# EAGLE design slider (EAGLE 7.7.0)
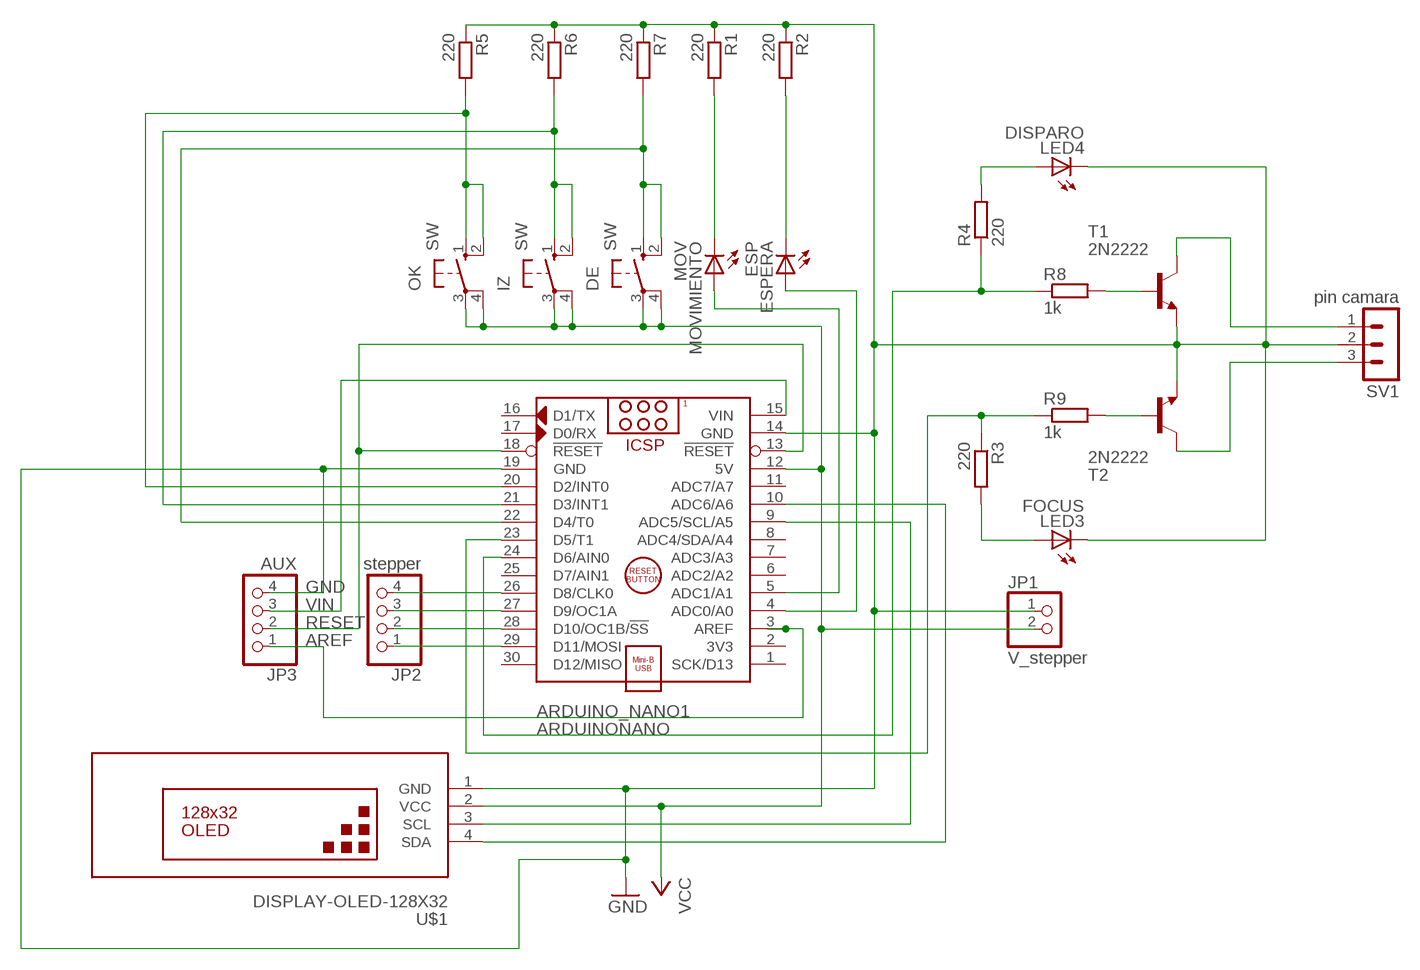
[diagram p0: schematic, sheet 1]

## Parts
ARDUINO_NANO1  ARDUINONANO  ARDUINO_NANO  [ARDUINO_NANO]
DE  SW  40-XX  [B3F-40XX]
ESPERA  ESP  LED5MM  [LED5MM]
IZ  SW  40-XX  [B3F-40XX]
JP1  V_stepper  PINHD-1X2  [1X02]
JP2  stepper  PINHD-1X4  [1X04]
JP3  AUX  PINHD-1X4  [1X04]
LED3  FOCUS  LED5MM  [LED5MM]
LED4  DISPARO  LED5MM  [LED5MM]
MOVIMIENTO  MOV  LED5MM  [LED5MM]
OK  SW  40-XX  [B3F-40XX]
R1  220  R-EU_0204/5  [0204/5]
R2  220  R-EU_0204/5  [0204/5]
R3  220  R-EU_0204/5  [0204/5]
R4  220  R-EU_0204/5  [0204/5]
R5  220  R-EU_0204/5  [0204/5]
R6  220  R-EU_0204/5  [0204/5]
R7  220  R-EU_0204/5  [0204/5]
R8  1k  R-EU_0204/5  [0204/5]
R9  1k  R-EU_0204/5  [0204/5]
SV1  pin camara  MA03-1  [MA03-1]
T1  2N2222  [TO92-EBC-OVAL]
T2  2N2222  [TO92-EBC-OVAL]
U$1  DISPLAY-OLED-128X32  [DISPLAY-OLED-128X32]

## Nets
AREF: ARDUINO_NANO1.3(AREF) JP3.1
GND: ARDUINO_NANO1.14(GND) ARDUINO_NANO1.19(GND) JP1.1 JP3.4 LED3.K(C) LED4.K(C) R1.1 R2.1 R5.1 R6.1 R7.1 SV1.2 T1.E T2.E U$1.1(GND)
N$1: ARDUINO_NANO1.24(D6/AIN0) R4.1 R8.1
N$2: ARDUINO_NANO1.29(D11/MOSI) JP2.1
N$3: ARDUINO_NANO1.28(D10/OC1B/!SS) JP2.2
N$4: ARDUINO_NANO1.27(D9/OC1A) JP2.3
N$5: MOVIMIENTO.K(C) R1.2
N$6: ESPERA.K(C) R2.2
N$7: ARDUINO_NANO1.22(D4/T0) DE.1(S) DE.2(S1) R7.2
N$8: R9.2 T2.B
N$9: R8.2 T1.B
N$10: LED4.A R4.2
N$12: ARDUINO_NANO1.4(ADC0/A0) ESPERA.A
N$13: LED3.A R3.2
N$14: SV1.3 T2.C
N$15: SV1.1 T1.C
N$16: ARDUINO_NANO1.23(D5/T1) R3.1 R9.1
N$17: ARDUINO_NANO1.5(ADC1/A1) MOVIMIENTO.A
N$18: ARDUINO_NANO1.21(D3/INT1) IZ.1(S) IZ.2(S1) R6.2
N$19: ARDUINO_NANO1.20(D2/INT0) OK.1(S) OK.2(S1) R5.2
N$21: ARDUINO_NANO1.9(ADC5/SCL/A5) U$1.3(SCL)
N$22: ARDUINO_NANO1.10(ADC6/A6) U$1.4(SDA)
N$23: ARDUINO_NANO1.26(D8/CLK0) JP2.4
RESET: ARDUINO_NANO1.13(!RESET) ARDUINO_NANO1.18(!RESET) JP3.2
VCC: ARDUINO_NANO1.12(5V) DE.3(P) DE.4(P1) IZ.3(P) IZ.4(P1) JP1.2 OK.3(P) OK.4(P1) U$1.2(VCC)
VIN: ARDUINO_NANO1.15(VIN) JP3.3
Unconnected: ARDUINO_NANO1.1(SCK/D13) ARDUINO_NANO1.2(3V3) ARDUINO_NANO1.6(ADC2/A2) ARDUINO_NANO1.7(ADC3/A3) ARDUINO_NANO1.8(ADC4/SDA/A4) ARDUINO_NANO1.11(ADC7/A7) ARDUINO_NANO1.16(D1/TX) ARDUINO_NANO1.17(D0/RX) ARDUINO_NANO1.25(D7/AIN1) ARDUINO_NANO1.30(D12/MISO)

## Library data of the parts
ARDUINO_NANO1 = ArduinoNanoV30:ARDUINO_NANO: Arduino Nano V3.0 Module Overview: The Arduino Nano is a small, complete, and breadboard-friendly board based on the ATmega328 (Arduino Nano 3.x) or ATmega168 (Arduino Nano 2.x). It has more or less the same functionality of the Arduino Duemilanove, but in a different package. It lacks only a DC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
DE IZ OK = switch-omron:40-XX: OMRON SWITCH; MF: OMRON COMPONENTS USA; MPN: B3F-4000; OC_FARNELL: 176434; OC_NEWARK: 36K3105
ESPERA LED3 LED4 MOVIMIENTO = adafruit:LED: LED
JP1 = pinhead:PINHD-1X2: PIN HEADER
JP2 JP3 = pinhead:PINHD-1X4: PIN HEADER
R1-R9 = rcl:R-EU_: RESISTOR, European symbol
SV1 = con-lstb:MA03-1: PIN HEADER; OC_FARNELL: unknown; OC_NEWARK: unknown
T1 T2 = adafruit:2N2222: NPN TRANSISTOR Big oval pads
U$1 = diy-modules:DISPLAY-OLED-128X32: 128x32 Dot Matrix OLED Module with I2C interface based on SSD1306 chip More details available here: http://www.tinyosshop.com/index.php?route=product/product&product_id=953 Schematic available here: http://www.tinyosshop.com/datasheet/OLED%2012832.pdf SSD1306 datasheet: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

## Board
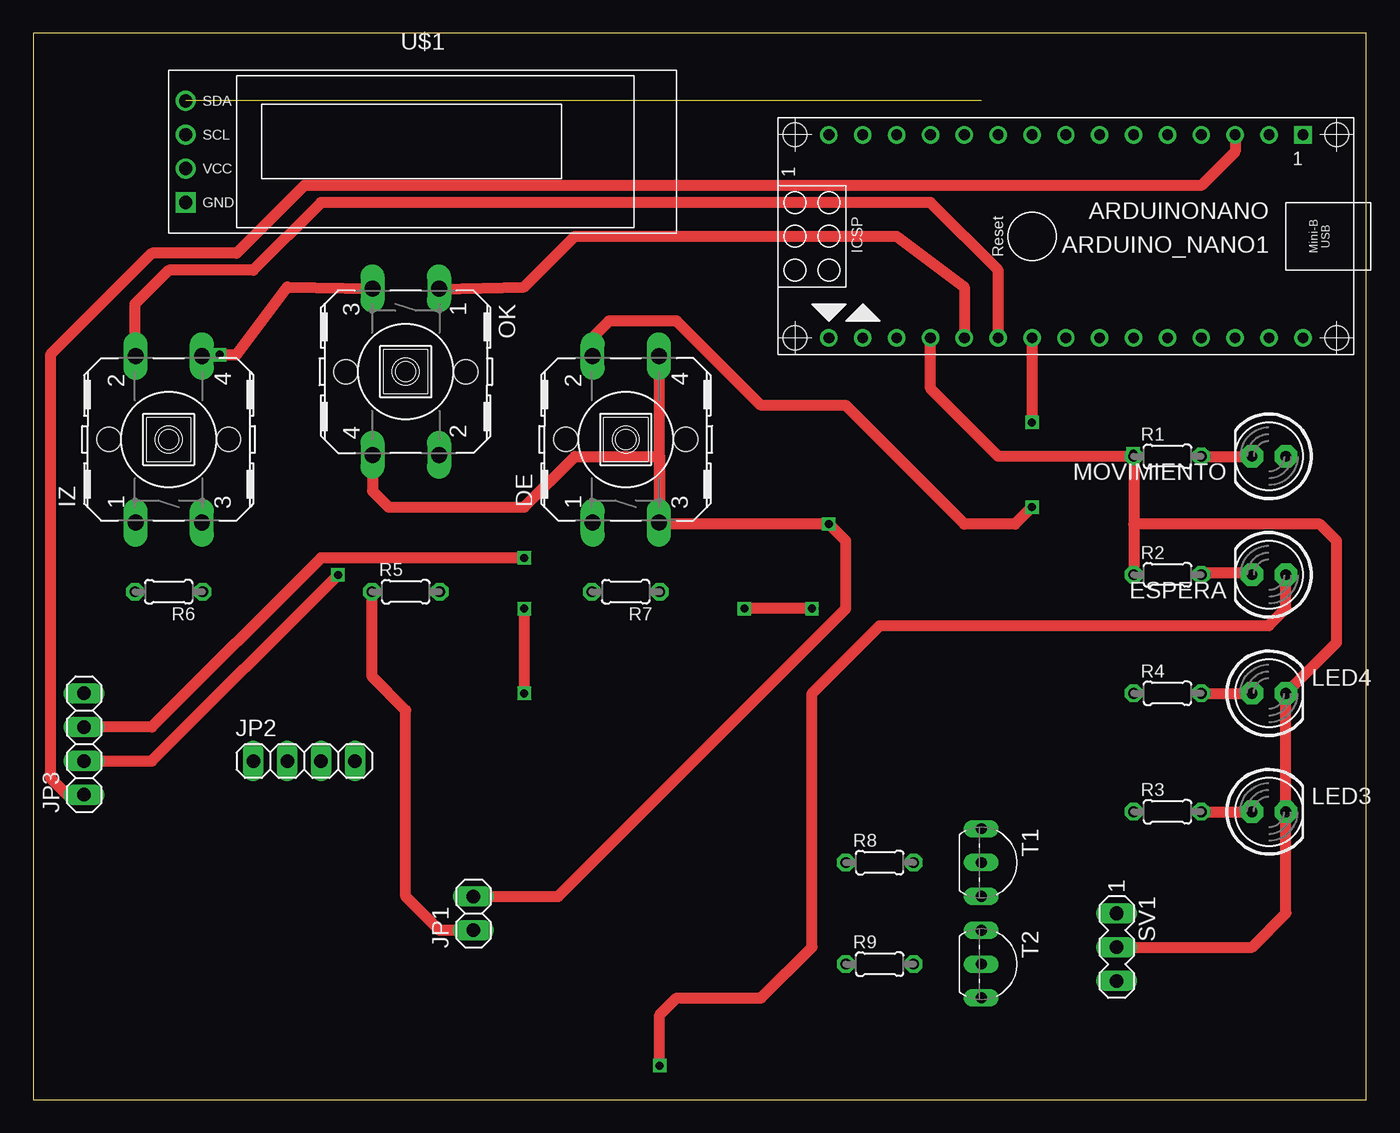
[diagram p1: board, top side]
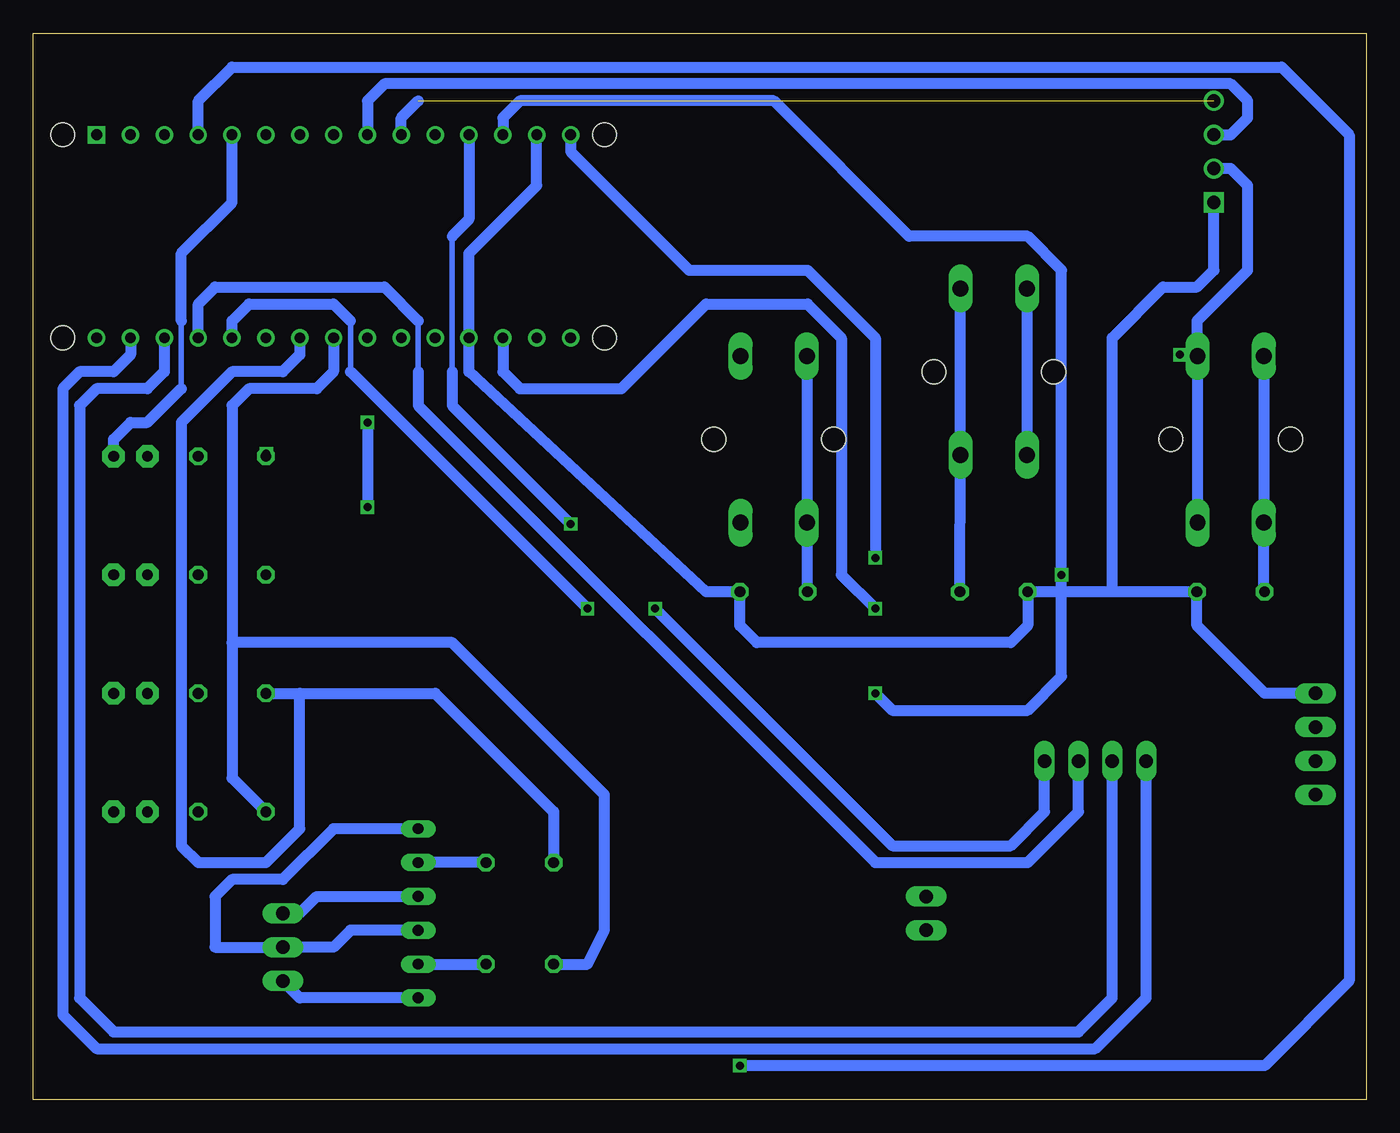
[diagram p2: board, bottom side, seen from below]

Size 100 x 80 mm. Coordinates in mm from the lower left corner, seen from the top.
Outline: 0,0 100,0 100,80 0,80 0,0
Copper layers (1*16): Top 0.035mm / dielectric 1.5mm / Bottom 0.035mm
Design rules "default": minimum track width 10mil, minimum drill 24mil, track to track 8mil, track to pad 8mil, pad to pad 8mil, via to via 8mil, smd to smd 8mil, copper to edge 40mil, drill to drill 8mil, minimum pad ring 10mil, minimum via ring 8mil, stop-mask expansion 4mil, vias tented up to drill 0mil, thermal gap 10mil

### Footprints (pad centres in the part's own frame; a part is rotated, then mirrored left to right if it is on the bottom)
ARDUINO_NANO = drill 0.8 square: 1 -20.32,-7.62 | drill 0.8: 2 -17.78,-7.62; 3 -15.24,-7.62; 4 -12.7,-7.62; 5 -10.16,-7.62; 6 -7.62,-7.62; 7 -5.08,-7.62; 8 -2.54,-7.62; 9 0,-7.62; 10 2.54,-7.62; 11 5.08,-7.62; 12 7.62,-7.62; 13 10.16,-7.62; 14 12.7,-7.62; 15 15.24,-7.62; 16 15.24,7.62; 17 12.7,7.62; 18 10.16,7.62; 19 7.62,7.62; 20 5.08,7.62; 21 2.54,7.62; 22 0,7.62; 23 -2.54,7.62; 24 -5.08,7.62; 25 -7.62,7.62; 26 -10.16,7.62; 27 -12.7,7.62; 28 -15.24,7.62; 29 -17.78,7.62; 30 -20.32,7.62 | hole 1.778: -22.86,-7.62; -22.86,7.62; 17.78,7.62; 17.78,-7.62
B3F-40XX = drill 1.194 long: 1 -6.248,2.489; 2 6.248,2.489; 3 -6.248,-2.489; 4 6.248,-2.489 | hole 1.803: 0,-4.496; 0,4.496
LED5MM = drill 0.813 pad 1.676 octagon: A -1.27,0; K 1.27,0
1X02 = drill 1.016 long: 1 -1.27,0; 2 1.27,0
1X04 = drill 1.016 long: 1 -3.81,0; 2 -1.27,0; 3 1.27,0; 4 3.81,0
0204/5 = drill 0.813 octagon: 1 -2.54,0; 2 2.54,0
MA03-1 = drill 1.016 long: 1 -2.54,0; 2 0,0; 3 2.54,0
TO92-EBC-OVAL = drill 0.813 long: B 0,-1.27; C 2.54,-1.27; E -2.54,-1.27
DISPLAY-OLED-128X32 = drill 1 square: 1 -17.78,-3.81 | drill 1: 2 -17.78,-1.27; 3 -17.78,1.27; 4 -17.78,3.81

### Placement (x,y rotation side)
ARDUINO_NANO1  74.93,64.77 180 top
DE  44.45,49.53 90 top
ESPERA  92.71,39.37 180 top
IZ  10.16,49.53 90 top
JP1  33.02,13.97 90 top
JP2  20.32,25.4 0 top
JP3  3.81,26.67 90 top
LED3  92.71,21.59 0 top
LED4  92.71,30.48 0 top
MOVIMIENTO  92.71,48.26 180 top
OK  27.94,54.61 270 top
R1  85.09,48.26 0 top
R2  85.09,39.37 0 top
R3  85.09,21.59 0 top
R4  85.09,30.48 0 top
R5  27.94,38.1 0 top
R6  10.16,38.1 180 top
R7  44.45,38.1 180 top
R8  63.5,17.78 0 top
R9  63.5,10.16 0 top
SV1  81.28,11.43 270 top
T1  72.39,17.78 270 top
T2  72.39,10.16 270 top
U$1  29.21,71.12 0 top

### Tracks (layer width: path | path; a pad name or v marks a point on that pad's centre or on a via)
AREF
  Top 0.813: ARDUINO_NANO1.3 90.17,71.12 87.63,68.58 20.32,68.58 15.24,63.5 8.89,63.5 1.27,55.88 1.27,24.13 2.54,22.86 JP3.1
GND  (via drill 0.6)
  Top 0.813: JP1.1 30.48,12.7 27.94,15.24 27.94,29.21 25.4,31.75 R5.1 | SV1.2 91.44,11.43 93.98,13.97 LED3.K LED4.K 97.79,34.29 97.79,41.91 96.52,43.18 82.55,43.18 R2.1 R1.1 | v82.53,48.46 82.32,48.26 72.39,48.26 67.31,53.34 ARDUINO_NANO1.19
  Bottom 0.254: v82.53,48.46 R1.1
  Bottom 0.813: 19.05,38.1 R5.1 25.4,35.56 26.67,34.29 45.72,34.29 46.99,35.56 R7.1 49.53,38.1 67.31,54.61 ARDUINO_NANO1.19 67.31,63.5 62.23,68.58 ARDUINO_NANO1.14 | 19.05,38.1 R6.1 12.7,35.56 7.62,30.48 JP3.4 | 19.05,38.1 19.05,57.15 15.24,60.96 12.7,60.96 11.43,62.23 U$1.1 | T2.E 76.2,12.7 77.47,11.43 SV1.2 86.36,11.43 86.36,15.24 85.09,16.51 81.28,16.51 77.47,20.32 T1.E
N$1
  Bottom 0.813: ARDUINO_NANO1.24 80.01,55.88 81.28,54.61 85.09,54.61 88.9,50.8 88.9,19.05 87.63,17.78 82.55,17.78 80.01,20.32 80.01,30.48 | R4.1 80.01,30.48 | 80.01,30.48 69.85,30.48 60.96,21.59 R8.1
N$2
  Bottom 0.813: ARDUINO_NANO1.29 92.71,55.88 93.98,54.61 96.52,54.61 97.79,53.34 97.79,6.35 95.25,3.81 20.32,3.81 16.51,7.62 JP2.1
N$3
  Bottom 0.813: ARDUINO_NANO1.28 90.17,54.61 91.44,53.34 95.25,53.34 96.52,52.07 96.52,7.62 93.98,5.08 21.59,5.08 19.05,7.62 JP2.2
N$4
  Bottom 0.406: 71.12,58.42 71.12,54.61
  Bottom 0.813: ARDUINO_NANO1.27 87.63,59.69 86.36,60.96 73.66,60.96 71.12,58.42 | 71.12,54.61 71.12,52.07 36.83,17.78 25.4,17.78 21.59,21.59 JP2.3
N$5
  Top 0.813: R1.2 MOVIMIENTO.K
N$6
  Top 0.254: 87.78,39.55 R2.2 | 91.44,39.55 ESPERA.K
  Top 0.813: 87.78,39.55 91.26,39.55 ESPERA.K
N$7  (via drill 0.6)
  Top 0.813: ARDUINO_NANO1.22 v74.93,50.8 | v74.93,44.45 73.66,43.18 69.85,43.18 60.96,52.07 54.61,52.07 48.26,58.42 43.18,58.42 41.91,57.15 41.91,55.83 DE.2
  Bottom 0.813: DE.2 DE.1 41.91,43.23 R7.2 | v74.93,50.8 v74.93,44.45
N$8
  Bottom 0.813: T2.B R9.2
N$9
  Bottom 0.813: R8.2 T1.B
N$10
  Top 0.813: R4.2 LED4.A
N$12  (via drill 0.6)
  Top 0.813: v46.99,2.54 46.99,6.35 48.26,7.62 54.61,7.62 58.42,11.43 58.42,30.48 63.5,35.56 92.71,35.56 93.98,36.83 ESPERA.A
  Bottom 0.813: ARDUINO_NANO1.4 87.63,74.93 85.09,77.47 6.35,77.47 1.27,72.39 1.27,8.89 7.62,2.54 v46.99,2.54
N$13
  Top 0.813: R3.2 LED3.A
N$14
  Bottom 0.813: T2.C 80.01,7.62 SV1.3
N$15
  Bottom 0.813: SV1.1 80.01,13.97 78.74,15.24 T1.C
N$16
  Bottom 0.813: ARDUINO_NANO1.23 77.47,54.61 78.74,53.34 83.82,53.34 85.09,52.07 85.09,34.29 | 85.09,34.29 85.09,24.13 R3.1 | R9.1 58.42,10.16 57.15,12.7 57.15,22.86 68.58,34.29 85.09,34.29
N$17
  Bottom 0.406: 88.9,53.34 88.9,58.42
  Bottom 0.813: MOVIMIENTO.A 93.98,49.53 92.71,50.8 91.44,50.8 88.9,53.34 | 88.9,58.42 88.9,63.5 85.09,67.31 ARDUINO_NANO1.5
N$18
  Top 0.813: ARDUINO_NANO1.21 72.39,62.23 67.31,67.31 21.59,67.31 16.51,62.23 10.16,62.23 7.62,59.69 7.62,55.73 | 7.62,54.61 7.62,55.73 | 7.62,55.73 IZ.2
  Bottom 0.813: R6.2 7.67,38.15 IZ.1 IZ.2
N$19  (via drill 0.6)
  Top 0.813: v30.48,60.81 36.83,60.96 40.64,64.77 64.77,64.77 69.85,60.96 ARDUINO_NANO1.20
  Bottom 0.813: OK.1 v30.48,60.81 30.48,48.36 | 30.48,48.26 30.48,48.36 | 30.48,48.36 OK.2 R5.2
N$21
  Bottom 0.813: U$1.3 10.16,72.39 8.89,73.66 8.89,74.93 10.16,76.2 73.66,76.2 74.93,74.93 ARDUINO_NANO1.9
N$22  (1 unrouted)
  Bottom 0.813: ARDUINO_NANO1.10 72.39,73.66 71.12,74.93
N$23  (via drill 0.6)
  Top 0.813: v58.42,36.83 v53.34,36.83
  Bottom 0.406: 76.2,58.42 76.2,54.61
  Bottom 0.813: ARDUINO_NANO1.26 85.09,58.42 83.82,59.69 77.47,59.69 76.2,58.42 | 76.2,54.61 v58.42,36.83 | v53.34,36.83 35.56,19.05 26.67,19.05 24.13,21.59 JP2.4
RESET  (via drill 0.6)
  Top 0.813: JP3.2 8.89,25.4 v22.86,39.37 | v36.83,36.83 v36.83,30.48
  Bottom 0.254: 64.92,57.15 ARDUINO_NANO1.18 | 64.92,72.24 ARDUINO_NANO1.13
  Bottom 0.813: ARDUINO_NANO1.13 64.77,73.66 63.5,74.93 44.45,74.93 34.29,64.77 25.4,64.77 22.86,62.23 v22.86,39.37 22.86,31.75 25.4,29.21 35.56,29.21 v36.83,30.48 | ARDUINO_NANO1.18 64.77,54.61 63.5,53.34 55.88,53.34 49.53,59.69 41.91,59.69 39.37,57.15 39.37,39.37 v36.83,36.83
VCC  (via drill 0.6)
  Top 0.813: v13.97,55.88 15.24,55.88 19.05,60.96 OK.3 | DE.4 46.94,48.26 | 46.94,48.26 DE.3 47.04,43.18 | OK.4 25.45,45.67 26.67,44.45 36.83,44.45 40.64,48.26 46.94,48.26 | 47.04,43.18 v59.69,43.18 60.96,41.91 60.96,36.83 39.37,15.24 JP1.2 | 46.94,48.26 46.99,48.26 46.99,43.18 47.04,43.18
  Bottom 0.406: 68.58,64.77 68.58,54.61
  Bottom 0.813: 12.7,55.88 12.7,55.83 IZ.4 IZ.3 | U$1.2 10.16,69.85 8.89,68.58 8.89,62.23 12.7,58.42 12.7,55.88 | OK.3 OK.4 | 12.7,55.88 v13.97,55.88 | ARDUINO_NANO1.12 67.31,66.04 68.58,64.77 | 68.58,54.61 68.58,52.07 v59.69,43.18
VIN  (via drill 0.6)
  Top 0.813: v36.83,40.64 21.59,40.64 8.89,27.94 JP3.3
  Bottom 0.813: ARDUINO_NANO1.15 59.69,71.12 50.8,62.23 41.91,62.23 36.83,57.15 v36.83,40.64

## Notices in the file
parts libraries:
diy-modules: Released under the Creative Commons Attribution 4.0 International License: http://creativecommons.org/licenses/by/4.0
